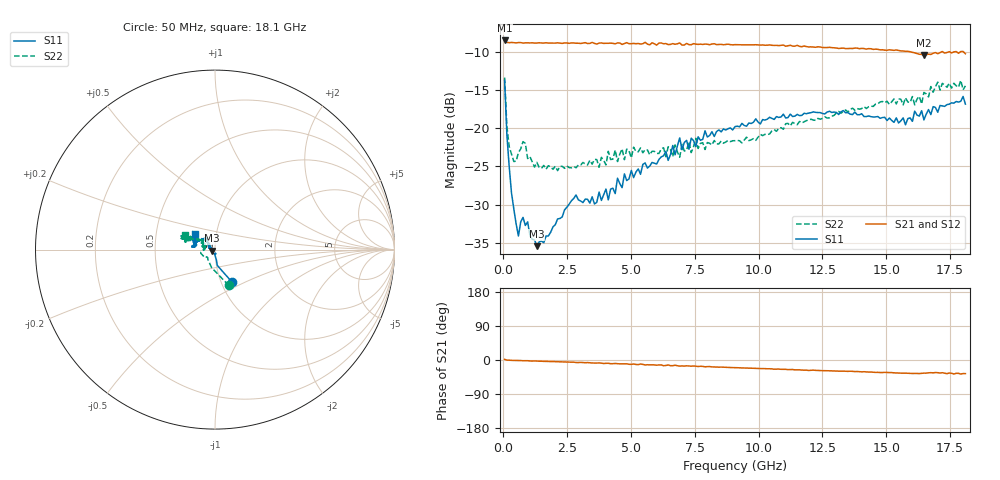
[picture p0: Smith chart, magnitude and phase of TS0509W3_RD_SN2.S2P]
! Network Analyzer HP8720D.06.14 Serial No. US36140669
! 30 Sep 2005  11:13:14
! Frequency  S11  S21  S12  S22
# HZ  S  DB R 50
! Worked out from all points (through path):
!   201 points, 50 MHz to 18.1 GHz, reference 50 ohm
!   highest |S21| = -8.55 dB at 50 MHz (marker M1); lowest = -10.5 dB at 16.48 GHz (marker M2)
!   group delay of S21, straight-line fit = 5.9 ps
!   lowest |S11| = -35.4 dB at 1.313 GHz (marker M3), VSWR 1.03, Z = 48.4 - j0.501 ohm
!   |S11| at or under -10 dB: start of sweep to end of sweep
!   |S22| runs from -25.6 to -13.4 dB; largest |S21 - S12| = 0.012
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5e7  -13.76 -62.3  -8.55 1.8  -8.56 2.0  -13.40 -69.0
1.4025e8  -20.98 -81.7  -8.80 -0.4  -8.77 -0.3  -19.81 -100.6
2.305e8  -25.05 -82.5  -8.84 -0.5  -8.82 -0.5  -22.44 -116.6
4.11e8  -30.56 -91.3  -8.84 -1.0  -8.83 -0.8  -24.36 -132.0
5.915e8  -34.10 -81.8  -8.82 -1.3  -8.83 -1.2  -23.20 -139.1
7.72e8  -31.67 -87.9  -8.89 -1.9  -8.84 -1.8  -21.77 -165.3
1.3135e9  -35.43 -162.2  -8.88 -3.0  -8.83 -2.7  -24.48 173.9
2.84775e9  -28.73 153.3  -8.91 -6.6  -8.88 -6.3  -25.18 151.1
3.1185e9  -29.73 164.5  -8.90 -6.8  -8.88 -6.9  -24.49 170.8
4.021e9  -27.97 151.5  -8.92 -8.7  -8.96 -8.4  -24.81 163.4
4.11125e9  -29.38 148.3  -8.92 -8.6  -8.84 -9.1  -23.04 164.0
4.47225e9  -26.54 138.5  -8.87 -9.8  -8.91 -9.2  -24.37 167.4
4.65275e9  -27.78 135.7  -9.07 -10.3  -8.89 -9.9  -22.71 167.2
6.09675e9  -24.08 135.3  -8.88 -13.0  -8.82 -13.0  -23.32 161.1
6.7285e9  -23.50 137.2  -9.05 -13.8  -9.08 -14.4  -22.20 153.1
6.909e9  -21.28 133.1  -8.87 -16.0  -8.99 -15.5  -23.80 150.0
7.54075e9  -22.43 132.0  -9.03 -16.3  -8.87 -16.7  -21.34 154.7
9.075e9  -19.80 149.3  -9.10 -20.2  -9.04 -20.0  -21.65 146.5
1.21435e10  -17.88 173.6  -9.41 -26.7  -9.36 -26.7  -18.95 151.4
1.512175e10  -18.68 169.1  -9.77 -33.2  -9.71 -32.4  -16.91 156.0
1.64755e10  -18.93 157.8  -10.46 -34.6  -10.32 -34.1  -15.34 156.4
1.81e10  -16.86 142.7  -10.29 -36.0  -10.24 -37.4  -14.48 153.6
